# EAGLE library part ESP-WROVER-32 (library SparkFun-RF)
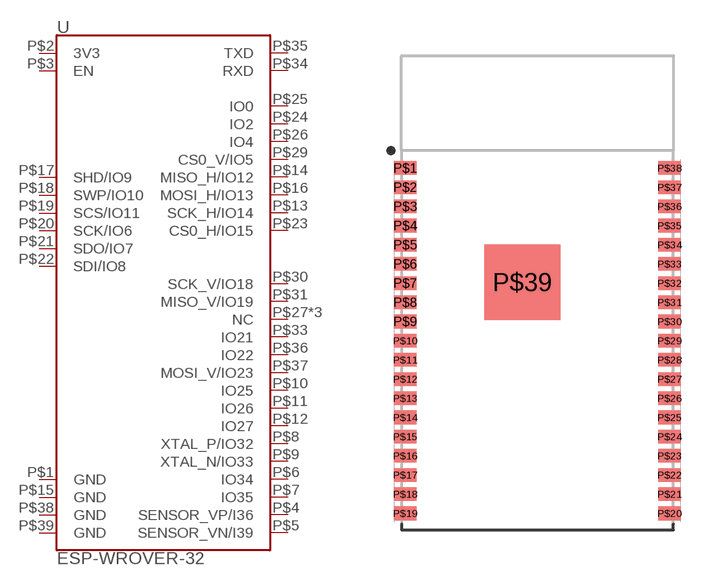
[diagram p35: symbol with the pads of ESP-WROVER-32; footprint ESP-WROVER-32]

Designator prefix U

## ESP-WROVER-32ESP-WROVER-32  [ESP-WROVER-32]
P$1  GND
P$2  3V3
P$3  EN
P$4  SENSOR_VP/I36
P$5  SENSOR_VN/I39
P$6  IO34
P$7  IO35
P$8  XTAL_P/IO32
P$9  XTAL_N/IO33
P$10  IO25
P$11  IO26
P$12  IO27
P$13  SCK_H/IO14
P$14  MISO_H/IO12
P$15  GND
P$16  MOSI_H/IO13
P$17  SHD/IO9
P$18  SWP/IO10
P$19  SCS/IO11
P$20  SCK/IO6
P$21  SDO/IO7
P$22  SDI/IO8
P$23  CS0_H/IO15
P$24  IO2
P$25  IO0
P$26  IO4
P$27  NC
P$28  NC
P$29  CS0_V/IO5
P$30  SCK_V/IO18
P$31  MISO_V/IO19
P$32  NC
P$33  IO21
P$34  RXD
P$35  TXD
P$36  IO22
P$37  MOSI_V/IO23
P$38  GND
P$39  GND

## Footprint ESP-WROVER-32 (pad centres in mm)
smd 1.5 x 0.9: P$1 0.25,-7.44; P$2 0.25,-8.71; P$3 0.25,-9.98; P$4 0.25,-11.25; P$5 0.25,-12.52; P$6 0.25,-13.79; P$7 0.25,-15.06; P$8 0.25,-16.33; P$9 0.25,-17.6; P$10 0.25,-18.87; P$11 0.25,-20.14; P$12 0.25,-21.41; P$13 0.25,-22.68; P$14 0.25,-23.95; P$15 0.25,-25.22; P$16 0.25,-26.49; P$17 0.25,-27.76; P$18 0.25,-29.03; P$19 0.25,-30.3; P$20 17.75,-30.3; P$21 17.75,-29.03; P$22 17.75,-27.76; P$23 17.75,-26.49; P$24 17.75,-25.22; P$25 17.75,-23.95; P$26 17.75,-22.68; P$27 17.75,-21.41; P$28 17.75,-20.14; P$29 17.75,-18.87; P$30 17.75,-17.6; P$31 17.75,-16.33; P$32 17.75,-15.06; P$33 17.75,-13.79; P$34 17.75,-12.52; P$35 17.75,-11.25; P$36 17.75,-9.98; P$37 17.75,-8.71; P$38 17.75,-7.44
smd 5 x 5: P$39 8,-15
